FUNCTION_BLOCK Delay // Delays rising edge propagation for a certain number of function block calls
VAR_INPUT
	Execute : BOOL; //Rising edge input
	Cycles : UDINT; //number of calls to delay for
END_VAR
VAR_OUTPUT
	Done : BOOL; //Ouput
END_VAR
VAR
	CyclesSinceRising : UDINT := 0;
END_VAR

IF Execute = FALSE THEN
	Done := FALSE;
	CyclesSinceRising := 0;
END_IF;

IF (Execute = TRUE) AND (CyclesSinceRising >= Cycles)THEN
	Done := TRUE;
END_IF; 

IF (Execute = TRUE) AND (Done = FALSE) THEN
	CyclesSinceRising := CyclesSinceRising + 1;
END_IF;

END_FUNCTION_BLOCK
